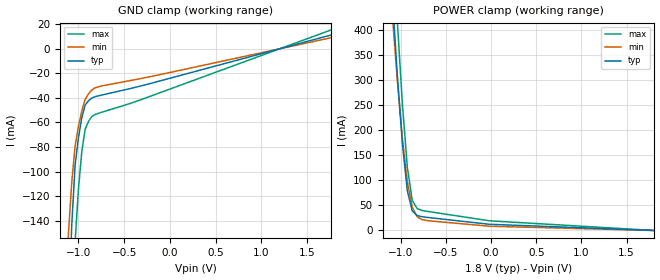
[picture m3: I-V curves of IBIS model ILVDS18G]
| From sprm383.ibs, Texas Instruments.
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|   Model ILVDS18G
[Model]   ILVDS18G
Model_type   Input
Polarity   Non-Inverting
Vinl =   0.5400V
Vinh =   1.2600V
C_comp   0.2879p   0.2833p   0.2907p
[Temperature Range]   25   105   0
[Voltage Range]   1.8   1.71   1.89
[POWER_clamp]
|   voltage   I(typ)   I(min)   I(max)
-1.8V     2.834A     2.412A     3.224A
-1.091V   461.2mA    424.9mA    592.1mA
-1.073V   409.8mA    382.4mA    532.8mA
-1.055V   358.5mA    339.8mA    473.6mA
-1.036V   307.1mA    297.3mA    414.3mA
-1.018V   262.7mA    259.8mA    360.6mA
-981.8mV  173.7mA    184.7mA    253.4mA
-927.3mV  79.54mA    97.47mA    126.7mA
-872.7mV  39.17mA    46.54mA    60.38mA
-818.2mV  29.78mA    27.26mA    43.53mA
-18.18mV  12.35mA    8.487mA    19.35mA
1.8V      0A         0A         0A
[GND_clamp]
|   voltage   I(typ)   I(min)   I(max)
-1.8V     -3.496A    -2.784A    -4.05A
-1.109V   -212.9mA   -150.1mA   -359.8mA
-1.073V   -142.9mA   -108.2mA   -246.9mA
-1.036V   -94.63mA   -79.02mA   -156.9mA
-1V       -72.47mA   -63.17mA   -114.2mA
-963.6mV  -56.22mA   -50.61mA   -83.77mA
-927.3mV  -45.88mA   -41.34mA   -65.61mA
-890.9mV  -42.39mA   -36.74mA   -59.26mA
-854.5mV  -40.1mA    -33.56mA   -55.21mA
-818.2mV  -38.99mA   -31.79mA   -53.47mA
-345.5mV  -30.8mA    -24.61mA   -42.2mA
1.764V    11.26mA    9.056mA    15.4mA
